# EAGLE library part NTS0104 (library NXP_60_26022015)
Dual supply translating transceiver; open drain; auto direction sensing The NTS0104 is a 4-bit, dual supply translating transceiver with auto direction sensing, that enables bidirectional voltage level translation. It features two 4-bit input-output ports (An and Bn), one output enable input (OE) and two supply pins (VCC(A) and VCC(B)). VCC(A) can be supplied at any voltage between 1.65 V and 3.6 V and VCC(B) can be supplied at any voltage between 2.3 V and 5.5 V, making the device suitable for translating between any of the voltage nodes (1.8 V, 2.5 V, 3.3 V and 5.0 V). Pins An and OE are referenced to VCC(A) and pins Bn are referenced to VCC(B). A LOW level at pin OE causes the outputs to assume a high-impedance OFF-state. This device is fully specified for partial power-down applications using IOFF. The IOFF circuitry disables the output, preventing the damaging backflow current through the device when it is powered down. AAL Eindhoven MK
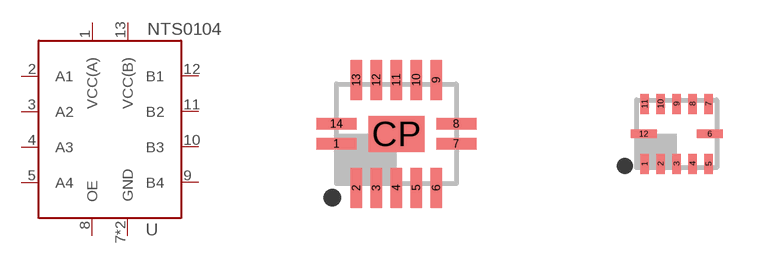
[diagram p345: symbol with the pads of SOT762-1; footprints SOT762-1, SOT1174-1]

Designator prefix U

## NTS0104BQ  [SOT762-1]
1  VCC(A)  out
2  A1  out
3  A2  out
4  A3  out
5  A4  out
7  GND  out
8  OE  out
9  B4  out
10  B3  out
11  B2  out
12  B1  out
13  VCC(B)  out
CP  GND  out

## NTS0104GU12  [SOT1174-1]
1  VCC(A)  out
2  A1  out
3  A2  out
4  A3  out
5  A4  out
6  GND  out
7  B4  out
8  B3  out
9  B2  out
10  B1  out
11  VCC(B)  out
12  OE  out

## NTS0104PW  [SOT402-1]
1  VCC(A)  out
2  A1  out
3  A2  out
4  A3  out
5  A4  out
7  GND  out
8  OE  out
10  B4  out
11  B3  out
12  B2  out
13  B1  out
14  VCC(B)  out

## Footprint SOT762-1 (pad centres in mm)
SOT762-1 DHVQFN14: plastic dual in-line compatible thermal enhanced very thin quad flat package; no leads; 14 terminals; body 2.5 x 3 x 0.85 mm JEDEC: MO-241 IEC: -- JEITA: --
smd 1 x 0.29: 1 -1.5,-0.25; 7 1.5,-0.25; 8 1.5,0.25; 14 -1.5,0.25
smd 0.29 x 1: 2 -1,-1.35; 3 -0.5,-1.35; 4 0,-1.35; 5 0.5,-1.35; 6 1,-1.35; 9 1,1.35; 10 0.5,1.35; 11 0,1.35; 12 -0.5,1.35; 13 -1,1.35
smd 1.4 x 0.9: CP 0,0

## Footprint SOT1174-1 (pad centres in mm)
SOT1174-1 XQFN12: plastic, extremely thin quad flat package; no leads;12 terminals; body 1.70 x 2.00 x 0.50 mm JEDEC: -- IEC: MO-288 JEITA: --
smd 0.22 x 0.5: 1 -0.8,-0.75; 2 -0.4,-0.75; 3 0,-0.75; 4 0.4,-0.75; 5 0.8,-0.75; 7 0.8,0.75; 8 0.4,0.75; 9 0,0.75; 10 -0.4,0.75; 11 -0.8,0.75
smd 0.65 x 0.22: 6 0.825,0; 12 -0.825,0

## Footprint SOT402-1 (pad centres in mm)
SOT402-1 TSSOP14: plastic thin shrink small outline package; 14 leads; body width 4.4 mm JEDEC: MO-153 IEC: ---
smd 0.6 x 1.35: 1 -2.05,-2.925; 7 2.05,-2.925; 8 2.05,2.925; 14 -2.05,2.925
smd 0.4 x 1.35: 2 -1.3,-2.925; 3 -0.65,-2.925; 4 0,-2.925; 5 0.65,-2.925; 6 1.3,-2.925; 9 1.3,2.925; 10 0.65,2.925; 11 0,2.925; 12 -0.65,2.925; 13 -1.3,2.925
